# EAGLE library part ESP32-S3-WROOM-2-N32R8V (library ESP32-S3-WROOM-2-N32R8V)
Check availability
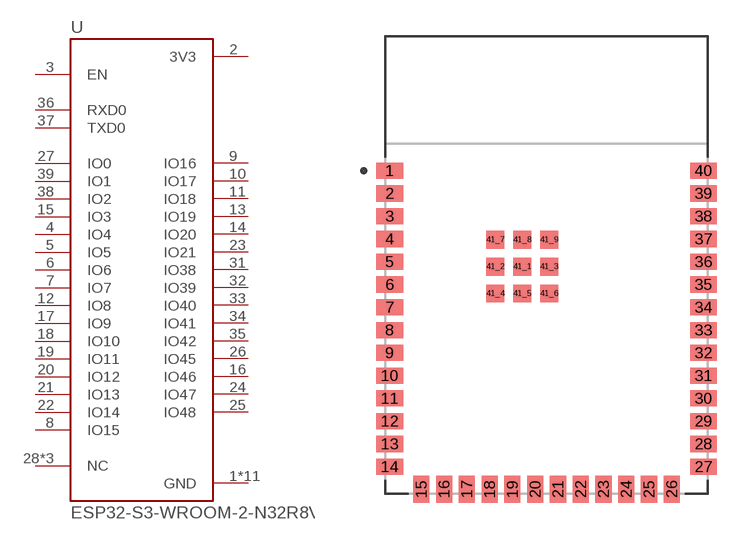
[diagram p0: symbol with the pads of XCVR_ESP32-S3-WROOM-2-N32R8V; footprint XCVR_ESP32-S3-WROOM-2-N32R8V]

Designator prefix U

## ESP32-S3-WROOM-2-N32R8V (AVAILABILITY: In Stock; DESCRIPTION: Bluetooth, WiFi 802.11b/g/n, Bluetooth v5.0 Transceiver Module 2.4GHz PCB Trace Surface Mount; MF: Espressif Systems; MP: ESP32-S3-WROOM-2-N32R8V; PACKAGE: Package; PRICE: None; PURCHASE-URL: https://pricing.snapeda.com/search/part/ESP32-S3-WROOM-2-N32R8V/?ref=eda)  [XCVR_ESP32-S3-WROOM-2-N32R8V]
1  GND  pwr
2  3V3  pwr
3  EN  in
4  IO4
5  IO5
6  IO6
7  IO7
8  IO15
9  IO16
10  IO17
11  IO18
12  IO8
13  IO19
14  IO20
15  IO3
16  IO46
17  IO9
18  IO10
19  IO11
20  IO12
21  IO13
22  IO14
23  IO21
24  IO47
25  IO48
26  IO45
27  IO0
28  NC  nc
29  NC  nc
30  NC  nc
31  IO38
32  IO39
33  IO40
34  IO41
35  IO42
36  RXD0
37  TXD0
38  IO2
39  IO1
40  GND  pwr
41_1  GND  pwr
41_2  GND  pwr
41_3  GND  pwr
41_4  GND  pwr
41_5  GND  pwr
41_6  GND  pwr
41_7  GND  pwr
41_8  GND  pwr
41_9  GND  pwr

## Footprint XCVR_ESP32-S3-WROOM-2-N32R8V (pad centres in mm)
smd 1.5 x 0.9: 1 -8.75,5.26; 2 -8.75,3.99; 3 -8.75,2.72; 4 -8.75,1.45; 5 -8.75,0.18; 6 -8.75,-1.09; 7 -8.75,-2.36; 8 -8.75,-3.63; 9 -8.75,-4.9; 10 -8.75,-6.17; 11 -8.75,-7.44; 12 -8.75,-8.71; 13 -8.75,-9.98; 14 -8.75,-11.25; 27 8.75,-11.25; 28 8.75,-9.98; 29 8.75,-8.71; 30 8.75,-7.44; 31 8.75,-6.17; 32 8.75,-4.9; 33 8.75,-3.63; 34 8.75,-2.36; 35 8.75,-1.09; 36 8.75,0.18; 37 8.75,1.45; 38 8.75,2.72; 39 8.75,3.99; 40 8.75,5.26
smd 0.9 x 1.5: 15 -6.985,-12.5; 16 -5.715,-12.5; 17 -4.445,-12.5; 18 -3.175,-12.5; 19 -1.905,-12.5; 20 -0.635,-12.5; 21 0.635,-12.5; 22 1.905,-12.5; 23 3.175,-12.5; 24 4.445,-12.5; 25 5.715,-12.5; 26 6.985,-12.5
smd 1 x 1: 41_1 -1.36,-0.09; 41_2 -2.86,-0.09; 41_3 0.14,-0.09; 41_4 -2.86,-1.59; 41_5 -1.36,-1.59; 41_6 0.14,-1.59; 41_7 -2.86,1.41; 41_8 -1.36,1.41; 41_9 0.14,1.41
